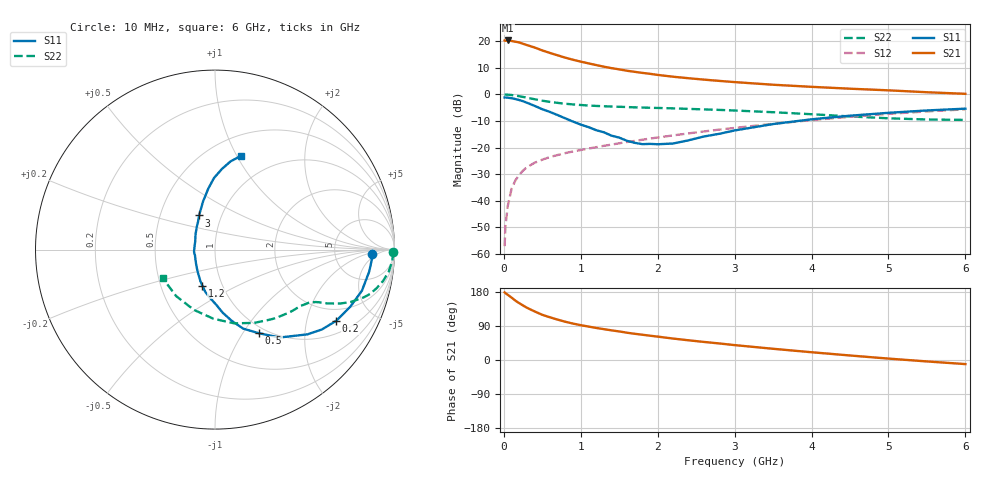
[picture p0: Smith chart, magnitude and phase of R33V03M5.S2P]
! SIEMENS Small Signal Semiconductors
! BFR181
! Si NPN RF Bipolar Junction Transistor in SOT23
! VCE = 3 V  IC = 3.5 mA
! Common Emitter S-Parameters:  May  1996
# GHz  S  MA  R  50
!  f  S11  S21  S12  S22
! GHz  MAG  ANG  MAG  ANG  MAG  ANG  MAG  ANG
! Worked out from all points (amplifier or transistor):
!   36 points, 10 MHz to 6 GHz, reference 50 ohm
!   highest |S21| = 20.3 dB at 50 MHz (marker M1)
!   |S21| within 3 dB of that: start of sweep to 431.5 MHz
!   unconditionally stable (mu >= 1): 1.28 GHz to 3.103 GHz
!   at 250 MHz: K = 0.33, MSG = 23.8 dB, |S12| = -28.6 dB
!   at 1.4 GHz: K = 1.03, MAG = 13.4 dB, |S12| = -18.9 dB
!   at 6 GHz: K = 0.85, MSG = 2.9 dB, |S12| = -5.6 dB
!   S11 on the Smith chart (normalised r, x): 10 MHz: 14, -3; 200 MHz: 1.47, -3.02; 500 MHz: 0.92, -1.19; 1.2 GHz: 0.80, -0.34; 3 GHz: 0.78, +0.31; 6 GHz: 0.70, +1.04
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0.01  0.8764 -1.7  10.33 178.4  0.0014 89.3  0.9944 -0.7
0.02  0.8762 -3.2  10.2 176.6  0.0032 91.9  0.993 -1.5
0.05  0.8682 -8.0  10.36 172.2  0.0079 86.8  0.9891 -3.7
0.1  0.8502 -15.6  10.14 164.8  0.0167 82.3  0.9758 -7.2
0.15  0.8181 -22.9  9.807 156.7  0.0242 77.4  0.9534 -10.5
0.2  0.7835 -30.4  9.497 150.0  0.0307 73.5  0.9261 -13.4
0.25  0.7439 -36.7  8.971 143.8  0.037 70.5  0.8982 -16.0
0.3  0.6989 -42.5  8.478 137.9  0.0427 68.6  0.8688 -17.9
0.4  0.609 -53.5  7.631 128.2  0.0519 64.8  0.8123 -21.0
0.5  0.5274 -62.2  6.724 119.2  0.0593 62.0  0.7623 -23.2
0.6  0.4679 -70.3  6.025 112.6  0.0666 60.8  0.7237 -24.5
0.8  0.3546 -83.0  4.911 100.9  0.0789 59.4  0.6684 -26.3
0.9  0.3083 -88.6  4.489 96.0  0.0847 59.3  0.6485 -26.9
1.1  0.2429 -102.7  3.843 88.3  0.0959 60.1  0.6191 -28.3
1.2  0.2128 -109.4  3.57 84.6  0.1017 60.3  0.6082 -28.9
1.6  0.1344 -141.1  2.791 72.0  0.1272 60.8  0.5797 -32.2
2.2  0.1194 157.4  2.154 56.6  0.1696 60.6  0.5469 -39.1
3  0.2101 115.0  1.707 39.3  0.2346 57.3  0.4984 -51.3
3.5  0.2773 103.8  1.522 29.6  0.28 53.8  0.463 -61.9
4.5  0.3982 90.9  1.282 11.9  0.3799 44.2  0.3855 -91.2
5.5  0.4999 79.9  1.1 -3.8  0.4794 31.6  0.3376 -129.9
6  0.5404 74.7  1.027 -10.8  0.5244 24.4  0.3318 -151.0
